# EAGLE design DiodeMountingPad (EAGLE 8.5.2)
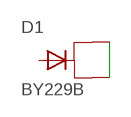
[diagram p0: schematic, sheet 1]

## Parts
D1  BY229B  [TO263AB]

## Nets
N$1: D1.1 D1.K
Unconnected: D1.2

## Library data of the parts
D1 = diode:BY229B: DIODE Fast Switching Rectifier, 8A (Vishay)

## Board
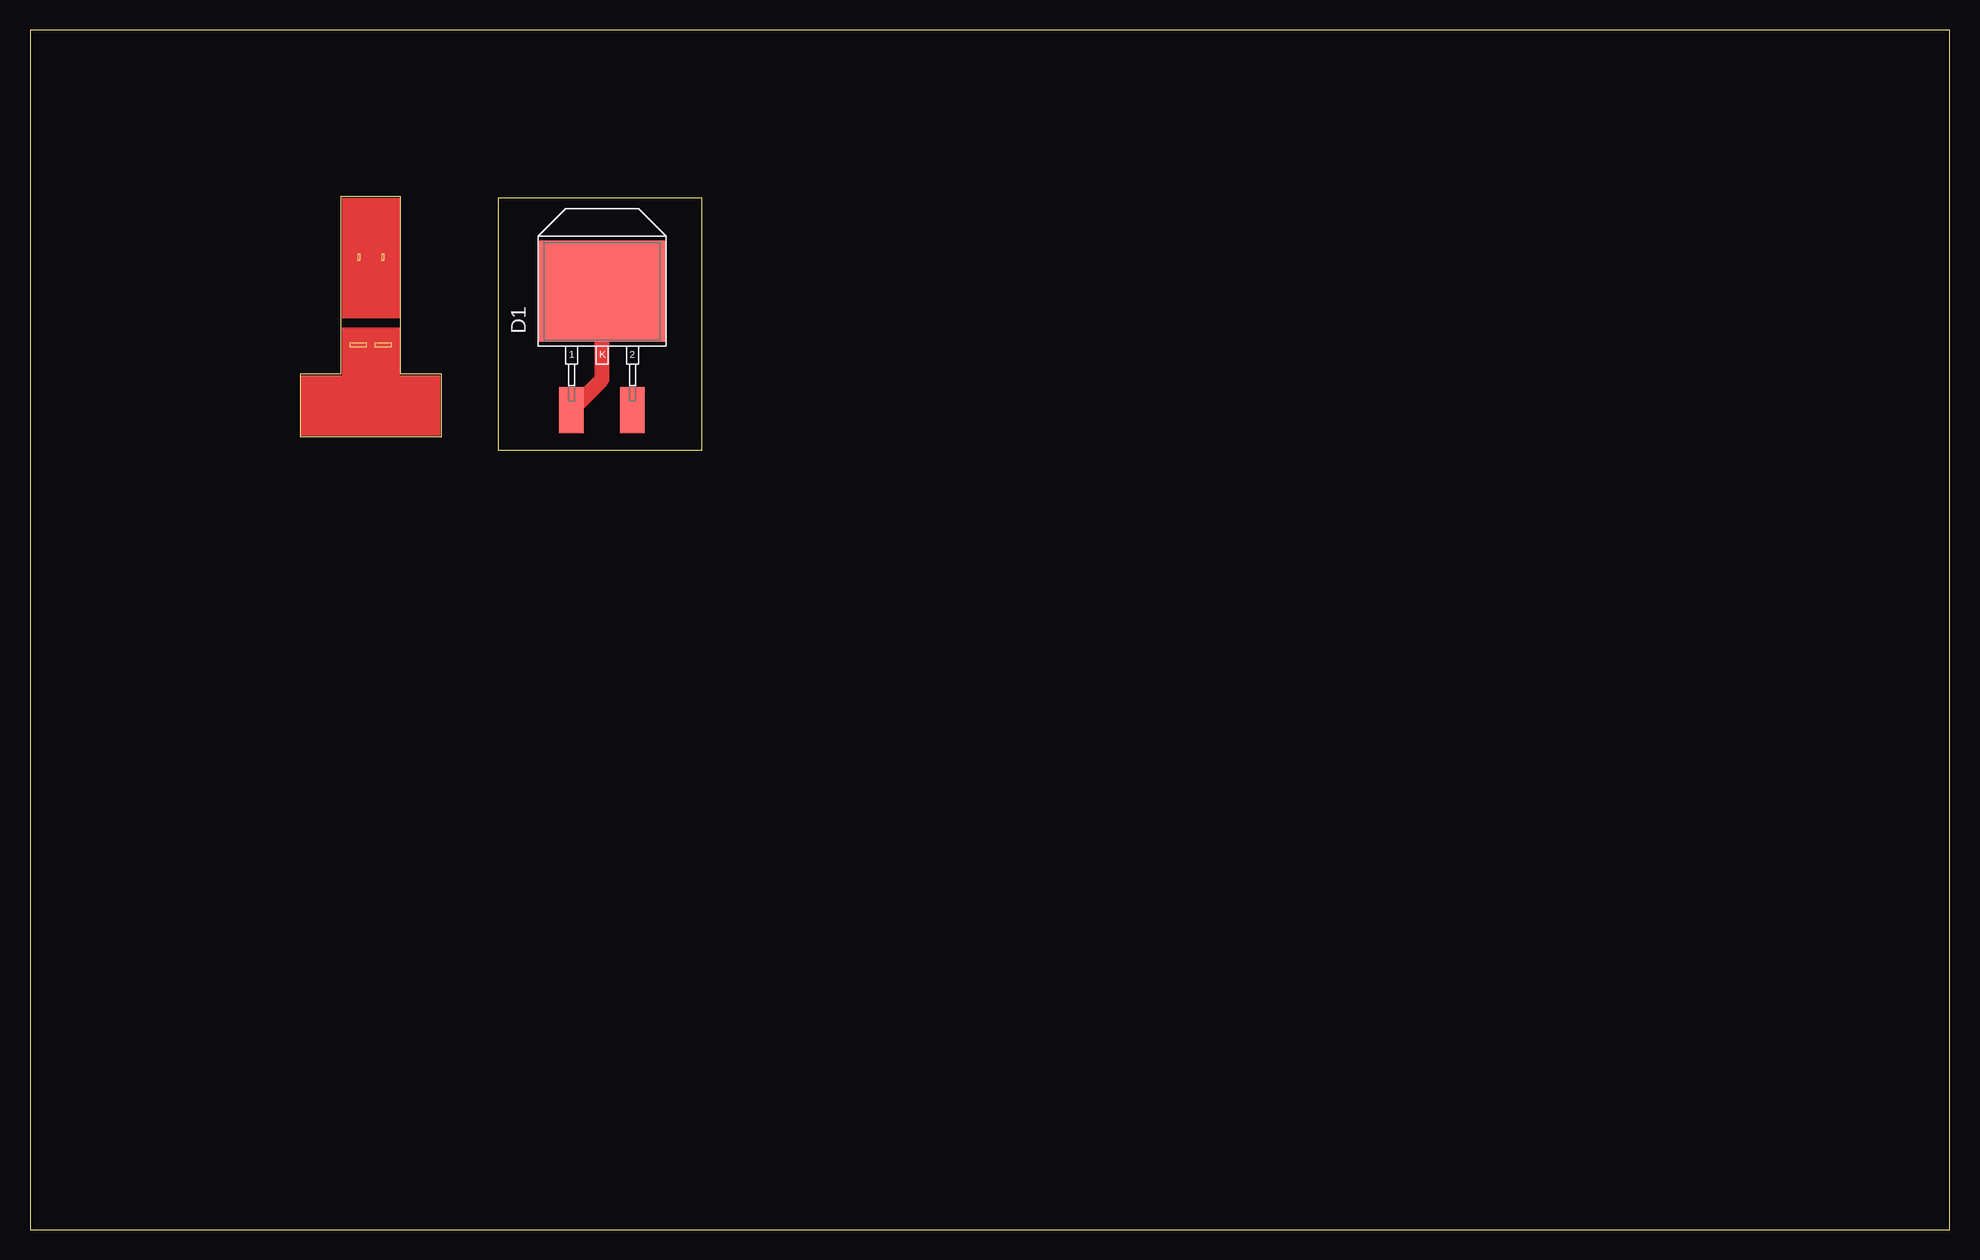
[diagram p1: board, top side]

Size 160 x 100 mm. Coordinates in mm from the lower left corner, seen from the top.
Outline: 0,0 160,0 160,100 0,100 0,0
Outline: 25.9,86.1 25.9,71.3 22.5,71.3 22.5,66.1 34.3,66.1 34.3,71.3 30.9,71.3 30.9,86.1 25.9,86.1
Copper layers (1*16): Top 0.035mm / dielectric 1.5mm / Bottom 0.035mm
Design rules "default": minimum track width 6mil, minimum drill 0.35mm, track to track 6mil, track to pad 6mil, pad to pad 6mil, via to via 6mil, smd to smd 6mil, copper to edge 40mil, drill to drill 6mil, minimum pad ring 10mil, minimum via ring 8mil, stop-mask expansion 4mil, vias tented up to drill 0mil, thermal gap 10mil
Milling: area 27.3,80.8 to 27.5,81.3; area 29.3,80.8 to 29.5,81.3; area 28.7,73.6 to 30.1,73.9; area 26.7,73.6 to 28.1,73.9

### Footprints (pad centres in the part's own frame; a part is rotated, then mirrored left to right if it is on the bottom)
TO263AB = smd 2.032 x 3.81: 1 -2.54,0; 2 2.54,0 | smd 10.668 x 8.382: K 0,9.906

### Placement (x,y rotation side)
D1  47.68,68.32 0 top

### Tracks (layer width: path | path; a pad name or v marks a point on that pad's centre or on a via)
N$1
  Top 1.27: D1.1 47.68,70.86 D1.K
(copper drawn outside any net)
  shapes: Top area x3

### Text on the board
Reference: Wire to rail | Bat Tab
